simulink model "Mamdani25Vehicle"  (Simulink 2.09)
settings: Solver=ode45  StartTime=0.0  StopTime=50  MaxStep=10  RelTol=1e-3  AbsTol=1e-3
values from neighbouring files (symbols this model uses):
  vd = 45    [VdataM.m]
undefined symbols (not defined in the file or in its folder): sfunyst
libraries: fuzzy x4

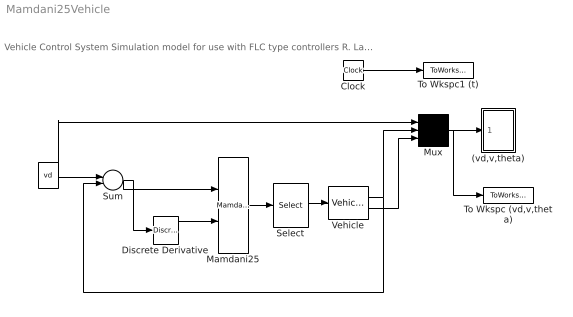
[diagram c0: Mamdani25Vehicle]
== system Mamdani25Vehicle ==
  note: Vehicle Control System Simulation model for use with FLC type controllers R. Langari 3/1/97
  " " : Constant  Value=vd
  (vd,v,theta) : Subsystem  mask(Storage scope.){}
      mask help: Storage scope using MATLAB graph window. Enter plotting ranges and line type.
      mask init:
      | npts = @4; color = @5; ax = [0, @1, @2, @3]; dt=-1;
  Clock : Clock
  Discrete Derivative : fuzzy/Discrete Derivative
  Mamdani25 : fuzzy/Mamdani25
  Mux : Mux  Inputs=3
  Select : fuzzy/Select
  Sum : Sum  Inputs=+-
  To Wkspc (vd,v,theta) : ToWorkspace  VariableName=yout  SampleTime=0
  To Wkspc1 (t) : ToWorkspace  VariableName=t  SampleTime=0
  Vehicle : fuzzy/Vehicle
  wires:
  Mux/1 -> To Wkspc (vd,v,theta)/1, (vd,v,theta)/1(x)
  Vehicle/1 -> Sum/2, Mux/2
  Vehicle/2 -> Mux/3
  Mamdani25/1 -> Select/1
  Select/1 -> Vehicle/1
  Clock/1 -> To Wkspc1 (t)/1
  Sum/1 -> Mamdani25/1, Discrete Derivative/1
  Discrete Derivative/1 -> Mamdani25/2
  " "/1 -> Sum/1, Mux/1

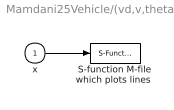
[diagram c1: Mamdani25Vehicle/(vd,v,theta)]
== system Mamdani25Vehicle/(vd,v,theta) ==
  x : Inport  Port=1  PortWidth=-1  SampleTime=-1
  "S-function M-file which plots lines " : S-Function  LoadFcn=sfunyst([],[],[],'LoadBlock')  FunctionName=sfunyst  Parameters=ax, color, npts, dt
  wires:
  x/1 -> "S-function M-file which plots lines "/1
